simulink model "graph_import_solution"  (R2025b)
settings: Solver=VariableStepAuto  StartTime=0.0  StopTime=10  RelTol=1e-3
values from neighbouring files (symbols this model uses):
  S = sum(round(C0))    [NormalizeCoef.m]
undefined symbols (not defined in the file or in its folder): AIE, AIE_Addition, class, code, Connector, Evaluation, file, FMC, graph_import, graph_import_ipconfig, Header, ML, netlist, Platform, tmp, VEK280, Versal, vmctmp, vsvh1760, Win_in_win_out, with, xcve2802
libraries: aieBasic x1, vmcUtilities x1, dspsrcs4 x1, aieUtilities x1

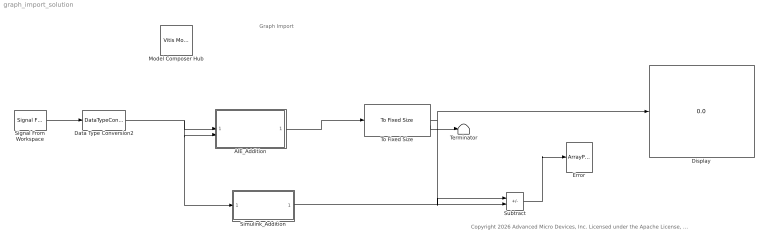
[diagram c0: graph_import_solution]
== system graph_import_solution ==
  note: Graph Import
  note: Copyright 2026 Advanced Micro Devices, Inc. Licensed under the Apache License, Version 2.0 (the "License"); you may not use this file except in compliance with the License. You may obtain a copy of the License at http://www.apache.org/licenses/LICENSE-2.0 Unless required by applicable law or agreed to in writing, software distributed under the License is distributed on an "AS IS" BASIS, WITHOUT WARRANTIES OR CONDITIONS OF ANY KIND, either express or implied. See the License for the specific language governing permissions and limitations under the License.
  AIE_Addition : Subsystem
  Data Type Conversion2 : DataTypeConversion  OutDataTypeStr=int16
  Display : Display
  Error : ArrayPlot  WindowPosition=[881.000000,237.000000,845.000000,423.000000,]  ScopeFrameLocation=window  PlotType=Line  ShowLegend=on
  Model Composer Hub : vmcUtilities/Vitis Model Composer Hub  Tag=genX  CodeGeneration=off  SubsystemName=AIE_Addition  BlockHierPath=graph_import/AIE_Addition  SubsystemType=AIENode  StartColumn=1  NumberOfColumns=1  TargetDirectory=./code  exportDesign=off  analyzeDesign=on  validateDesignOnHw=off  ExportType=AI Engines  IpVendor=xilinx.com  IpLibrary=hls  IpVersion=1.0  IpHWLanguage=Verilog  AieCompilerOptions={}  AieSimulatorOptions={}  CreateTestbench=on  TestbenchStackSize=10  RunRtlSim=off  RunCSim=off  RunAieSim=on  AieSimTimeout=50000  RunAieSimProfiling=off  LaunchVitisAnalyzer=off  PlotOutput=off  RunX86Sim=off  X86SimTimeout=10  GenHwImage=off  GenLibadfXo=off  GenHwValidationCode=off  PlatformType=Specify Platform  Platform=/opt/amd/2025.2/Vitis/base_platforms/xilinx_vek280_base_202520_1/xilinx_vek280_base_202520_1.xpfm  HwSystemType=Baremetal  HwValidationTarget=hw  ProjDevice=Versal VEK280 Evaluation Platform with FMC Connector (xcve2802-vsvh1760-2MP-e-S)  ProjDevicePart=xcve2802-vsvh1760-2MP-e-S  AIEType=AIE-ML  SamplePeriod=-1  ClockFrequency=200  DataPathParallelism=1  xilinxfamily=versalaiedge  part=xcve2802  speed=-2MP-e-S  package=vsvh1760  directory=./netlist  testbench=off  incr_netlist=off  synthesis_tool=Vivado  clock_wrapper=Clock Enables  dbl_ovrd=According to Block Masks  dcm_input_clock_period=10  sysclk_period=10  simulink_period=1  eval_field=0  IPInfoJsonString="{\"DUTSubsystemName\":\"AIE_Addition\",\"AIESubsystem\":{\"SubsystemName\":\"AIE_Addition\",\"TargetDirectory\":\"./code\",\"AIEArrayConfig\":\"Use entire AIE array\",\"StartColumn\":\"0\",\"NumberOfColumns\":\"1\"},\"SubsystemTag\":\"AIENode\"}"  LogFileName=/home/amd/training/Import_AIE_graph/lab/code/model_composer.log  NThreads=4  IPConfigFile=/tmp/vmctmp-3173931821410892050/graph_import_ipconfig.json
  Signal From Workspace : dspsrcs4/Signal From Workspace  X=1:16  Ts=1  nsamps=16  OutputAfterFinalValue=Setting to zero  ignoreOrWarnInputAndFrameLengths=off  OutputFrames=off
  Simulink_Addition : Subsystem
  Subtract : Sum  Inputs=+-
  Terminator : Terminator
  To Fixed Size : aieUtilities/To Fixed Size  Mode=Produce a valid output signal  OutputSize=Inherit: Same as input  CopyMethod=Buffer samples to form output  HasStatusOutput=on
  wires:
  To Fixed Size/1 -> Subtract/1, Display/1
  Signal From Workspace/1 -> Data Type Conversion2/1
  Simulink_Addition/1(Out1) -> Subtract/2
  Subtract/1 -> Error/1
  Data Type Conversion2/1 -> AIE_Addition/1(In1), AIE_Addition/2(In2), Simulink_Addition/1(In1)
  To Fixed Size/2 -> Terminator/1
  AIE_Addition/1(Out1) -> To Fixed Size/1

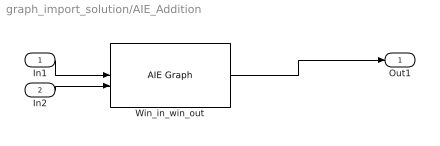
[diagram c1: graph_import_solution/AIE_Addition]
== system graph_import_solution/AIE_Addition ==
  In1 : Inport
  In2 : Inport  Port=2
  Win_in_win_out : aieBasic/AIE Graph  PortAttributesTable={'Input', 'In1', 'buffer', 'int16', '16', 'sync', '';'Input', 'In2', 'buffer', 'int16', '16', 'sync', '';'Output', 'Out1', 'buffer', 'int16', '16', 'sync', ''}  PortAttributesEnablement={'off', 'on', 'off', 'off', 'off', 'off', 'off';'off', 'on', 'off', 'off', 'off', 'off', 'off';'off', 'on', 'off', 'off', 'off', 'off', 'off'}  SampleTime=-1  ClassDeclTypeOptions=C[1 1]@t20@class Win_in_win_out  ClassDecl=class Win_in_win_out  ClassTemplateParams={}  ClassTemplateParamsEnables={}  ClassCtorDeclTypeOptions=C[1 1]@t7@<empty>  ClassCtorDecl=<empty>  ClassCtorParams={}  GraphAllAttrs=s[12;12;9;9;19;14;21;23;21;23;24;21;15;17;12;24;26;26;26;27;28;9;21;23;23;23;24;25;14;19;19;29]@FunctionNameDeclFileNamePortNamesPortTypesPortSerializedTypesPortDirectionsPortWindowSizeEnablesPortWindowMarginEnablesPortBufferSizeEnablesPortBufferMarginEnablesPortSynchronicityEnablesPortSignalSizeEnablesPortBufferSizesPortBufferMarginsFunctionDeclFunctionTemplateSpecKindFunctionTemplateParamNamesFu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  PortArgDecls={'in buffer int16 in1'; 'in buffer int16 in2'; 'out buffer int16 out1'}  PortGraphPortNames={'In1'; 'In2'; 'Out1'}  HierGraphPortNames={'In1'; 'In2'; 'Out1'}  PortTypes={'buffer'; 'buffer'; 'buffer'}  PortDataTypes={'int16'; 'int16'; 'int16'}  PortSizes={1.600000000000000000e+01; 1.600000000000000000e+01; 1.600000000000000000e+01}  PortSynchronicities={'sync'; 'sync'; 'sync'}  PortSignalSizes={0.000000000000000000e+00; 0.000000000000000000e+00; 0.000000000000000000e+00}  SimLibPath=''  ClassIndex=1  ClassCtorIndex=0  ClassTabVisible=off  FunctionTabVisible=on  DelayDrawLabels=off  GraphFileSelect=Header file (*.h)  GraphHeaderFile=win_in_win_out.h  GraphClassName=Win_in_win_out  GraphName=Win_in_win_out  GraphHeaderFiles={'./win_in_win_out.h'}  GraphSourceFile=./model_composer_work/xmc_aie_lib/25c7b9d7/mygraph.cpp  GraphSearchPaths={'./src/kernels'}  GraphPreProcOptions={}  blockJsonConstraints=[]
  Out1 : Outport
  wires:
  In1/1 -> Win_in_win_out/1
  In2/1 -> Win_in_win_out/2
  Win_in_win_out/1 -> Out1/1

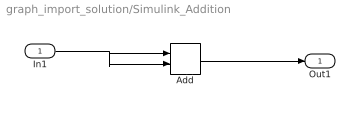
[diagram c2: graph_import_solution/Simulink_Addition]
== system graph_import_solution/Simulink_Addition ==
  In1 : Inport
  Add : Sum
  Out1 : Outport
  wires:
  In1/1 -> Add/2, Add/1
  Add/1 -> Out1/1
